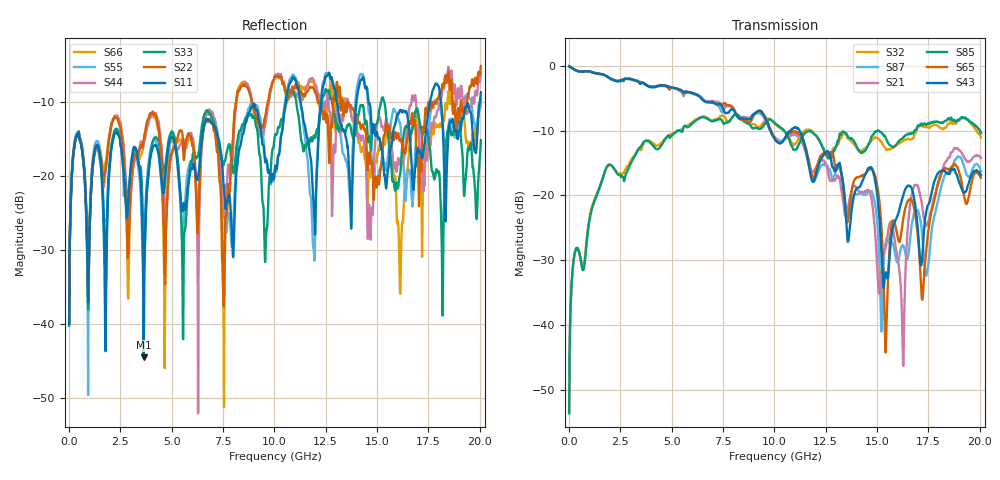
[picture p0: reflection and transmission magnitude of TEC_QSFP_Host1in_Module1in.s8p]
!!  This file represents Tyco Electronics parts only.  Due to internal design and materials, it should not  !!
!!  be used for products manufactured by companies other than Tyco Electronics.  !!
!! FILE NAME: TEC_QSFP_Host1in_Module1in.s8p
!! PART DESCRIPTION: Tyco Electronics QSFP P/N 1761987-9
!! PCB DESCRIPTION: Host Board FR4 with 1.5 inch microstrip, Module Board FR4 with 1.5 inch microstrip
!! FILE DESCRIPTION: 8 Port, S-Parameter, Measured Channel
!! FILE REVISION: Revision 2, 3/11/2008
!! FILE FREQUENCY RANGE: DC to 20.05 GHz in 12.50 MHz frequency steps
!! PORT DEFINITIONS:
!! Port  1  ----->  Host	Pin 24, RX4-	Module  <-----  Port  2
!! Port  3  ----->  Host	Pin 25, RX4+	Module  <-----  Port  4
!! Port  5  ----->  Host	Pin 33, TX3+	Module  <-----  Port  6
!! Port  7  ----->  Host	Pin 34, TX3-	Module  <-----  Port  8
# HZ S MA R 50.00
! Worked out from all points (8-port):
!   1604 points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, 12.5 MHz to 20.05 GHz, reference 50 ohm
!   strongest paths, dB at 12.5 MHz, 5.025 GHz, 10.04 GHz, 15.05 GHz, 20.05 GHz:
!     S43: -0.1, -3.4, -11.4, -21.2, -16.9
!     S65: -0.1, -3.4, -11.3, -19.3, -17.3
!     S85: -53.7, -10.7, -8.9, -10.0, -10.4
!     S21: 0.0, -3.4, -11.2, -33.6, -14.2
!     S87: -0.1, -3.4, -11.1, -26.0, -16.3
!     S32: -53.5, -10.5, -9.0, -11.2, -11.0
!   lowest |S11| = -44.5 dB at 3.638 GHz (marker M1), VSWR 1.01, Z = 50.6 - j0.112 ohm
!   |S11| at or under -10 dB: start of sweep to 10.55 GHz; 14.59 GHz to 17.58 GHz (2.992 GHz wide, 18.6 % of centre); 18.11 GHz to 20 GHz (1.886 GHz wide, 9.9 % of centre)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
